{attribute 'no_assign'}
FUNCTION_BLOCK FB_LN_IED_MUnn_InnATCTR1 EXTENDS FB_AcsiCommonLogicalNodeClass
VAR_INPUT
	Beh: FB_DO_IED_MUnn_InnATCTR1_Beh := (sClass:='ENS', bLinkResult:=THIS^.AddDataToContainer(ipData:=Beh));
	AmpSv: FB_DO_IED_MUnn_InnATCTR1_AmpSv := (sClass:='SAV', bLinkResult:=THIS^.AddDataToContainer(ipData:=AmpSv)); (*Current (sampled value)*)
END_VAR
VAR
END_VAR

END_FUNCTION_BLOCK
